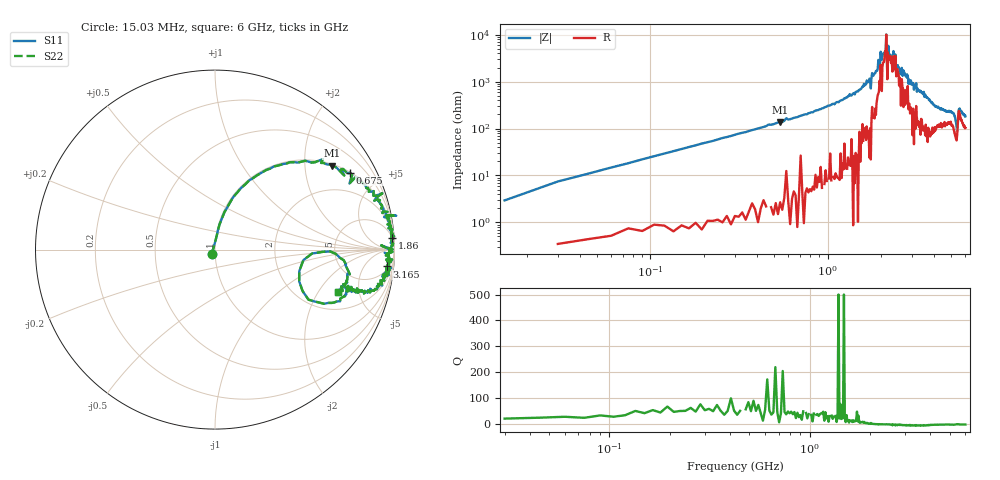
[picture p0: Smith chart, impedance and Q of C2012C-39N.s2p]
!	Network	Analyzer	HP8753E.07.74:	Oct	30	2002	Serial	No.	JP38451487
!	Hewlett-Packard
!	7	Sep	2009	10:54:08
!	Frequency	S11	S21	S12	S22
#	HZ	S	RI	R	50
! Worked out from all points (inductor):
!   400 points, 15.03 MHz to 6 GHz, reference 50 ohm
!   read as one part in series: L = 39 nH near 45.03 MHz
!   highest Q = 55.4 at 540 MHz (marker M1), where L = 40.5 nH
!   self-resonance near 2.184 GHz
!   S11 on the Smith chart (normalised r, x): 15.03 MHz: 0.97, -0.05; 675 MHz: 1.02, +3.50; 1.86 GHz: 6, +30; 3.165 GHz: 7, -18; 6 GHz: 3.05, -3.04
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1.502992e7  -0.0171 -0.0235  1.02 0.0235  1.02 0.0235  -0.0171 -0.0235
6.00297e7  0.0263 0.143  0.974 -0.143  0.974 -0.143  0.0263 0.143
1.500292e8  0.124 0.318  0.876 -0.318  0.876 -0.318  0.124 0.318
5.400273e8  0.651 0.467  0.349 -0.467  0.349 -0.467  0.651 0.467
6.750266e8  0.753 0.429  0.247 -0.429  0.247 -0.429  0.753 0.429
1.020025e9  0.898 0.289  0.102 -0.289  0.102 -0.289  0.898 0.289
1.860021e9  0.985 0.0629  0.0154 -0.0629  0.0154 -0.0629  0.985 0.0629
2.01002e9  0.986 0.0301  0.0137 -0.0301  0.0137 -0.0301  0.986 0.0301
2.130019e9  0.979 0.0076  0.0207 -0.0076  0.0207 -0.0076  0.979 0.0076
2.145019e9  0.99 0.00137  0.00967 -0.00137  0.00967 -0.00137  0.99 0.00137
2.175019e9  0.926 0.0235  0.0742 -0.0235  0.0742 -0.0235  0.926 0.0235
2.205019e9  0.989 -0.0134  0.0105 0.0134  0.0105 0.0134  0.989 -0.0134
2.325018e9  0.964 -0.0278  0.0365 0.0278  0.0365 0.0278  0.964 -0.0278
2.355018e9  0.983 -0.0136  0.0172 0.0136  0.0172 0.0136  0.983 -0.0136
2.445018e9  0.952 -0.0334  0.0485 0.0334  0.0485 0.0334  0.952 -0.0334
3.015015e9  0.981 -0.103  0.0189 0.103  0.0189 0.103  0.981 -0.103
3.165014e9  0.957 -0.094  0.043 0.094  0.043 0.094  0.957 -0.094
4.00501e9  0.849 -0.241  0.151 0.241  0.151 0.241  0.849 -0.241
5.010005e9  0.741 -0.22  0.259 0.22  0.259 0.22  0.741 -0.22
5.385003e9  0.469 -0.176  0.531 0.176  0.531 0.176  0.469 -0.176
5.520002e9  0.73 -0.0831  0.27 0.0831  0.27 0.0831  0.73 -0.0831
6e9  0.684 -0.237  0.316 0.237  0.316 0.237  0.684 -0.237
